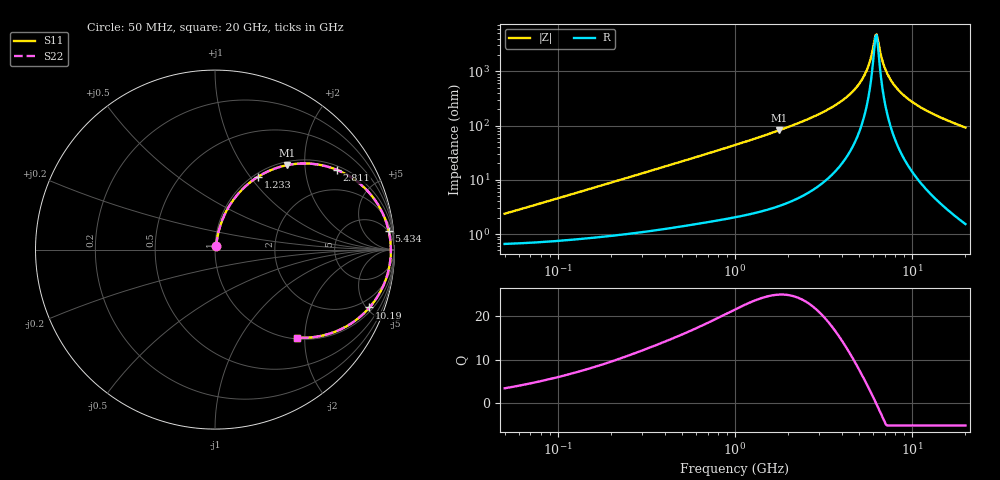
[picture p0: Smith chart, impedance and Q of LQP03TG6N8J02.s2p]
!Murata Part Number: LQP03TG6N8J02
!These Parameters are Measured in Series Mode Connection
!  o--[Z]--o
!Port1  Port2
!  o-------o
!Freq. Start=50[MHz] Stop=20[GHz], 401[Steps]
# Hz S RI R 50
!Freq.(Hz) S11(Real) S11(Imag) S21(Real) S21(Imag) S12(Real) S12(Imag) S22(Real) S22(Imag)
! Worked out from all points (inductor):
!   401 points, 50 MHz to 20 GHz, reference 50 ohm
!   read as one part in series: L = 7.23 nH near 51.52 MHz
!   highest Q = 24.8 at 1.767 GHz (marker M1), where L = 7.31 nH
!   self-resonance near 6.218 GHz
!   S11 on the Smith chart (normalised r, x): 50 MHz: 1.01, +0.05; 1.233 GHz: 1.05, +1.09; 2.811 GHz: 1.14, +2.96; 5.434 GHz: 4, +18; 10.19 GHz: 1.26, -5.22; 20 GHz: 1.03, -1.84
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5e7  0.00706 0.0225  0.9929 -0.0225  0.9929 -0.0225  0.00706 0.0225
1.364002e8  0.0117 0.0598  0.9883 -0.0598  0.9883 -0.0598  0.0117 0.0598
3.721004e8  0.0367 0.1547  0.9633 -0.1547  0.9633 -0.1547  0.0367 0.1547
1e9  0.1717 0.3545  0.8283 -0.3545  0.8283 -0.3545  0.1717 0.3545
1.23331e9  0.2384 0.405  0.7616 -0.405  0.7616 -0.405  0.2384 0.405
1.766834e9  0.4011 0.4704  0.5989 -0.4704  0.5989 -0.4704  0.4011 0.4704
2.728004e9  0.6613 0.4513  0.3387 -0.4513  0.3387 -0.4513  0.6613 0.4513
2.810964e9  0.6798 0.4441  0.3202 -0.4441  0.3202 -0.4441  0.6798 0.4441
3.572216e9  0.8183 0.3577  0.1817 -0.3577  0.1817 -0.3577  0.8183 0.3577
4.275624e9  0.9011 0.2615  0.0989 -0.2615  0.0989 -0.2615  0.9011 0.2615
4.89267e9  0.9456 0.1757  0.0544 -0.1757  0.0544 -0.1757  0.9456 0.1757
5.433528e9  0.968 0.1034  0.032 -0.1034  0.032 -0.1034  0.968 0.1034
5.769027e9  0.9756 0.0606  0.0244 -0.0606  0.0244 -0.0606  0.9756 0.0606
6.125241e9  0.9794 0.0173  0.0206 -0.0173  0.0206 -0.0173  0.9794 0.0173
6.311513e9  0.9799 -0.00442  0.0201 0.00442  0.0201 0.00442  0.9799 -0.00442
6.406762e9  0.9797 -0.0153  0.0203 0.0153  0.0203 0.0153  0.9797 -0.0153
6.905011e9  0.9754 -0.0695  0.0246 0.0695  0.0246 0.0695  0.9754 -0.0695
7.442007e9  0.965 -0.1229  0.035 0.1229  0.035 0.1229  0.965 -0.1229
8.516016e9  0.9316 -0.2147  0.0684 0.2147  0.0684 0.2147  0.9316 -0.2147
1.019291e10  0.8606 -0.3226  0.1394 0.3226  0.1394 0.3226  0.8606 -0.3226
1.417136e10  0.6747 -0.4553  0.3253 0.4553  0.3253 0.4553  0.6747 -0.4553
2e10  0.4587 -0.49  0.5413 0.49  0.5413 0.49  0.4587 -0.49
